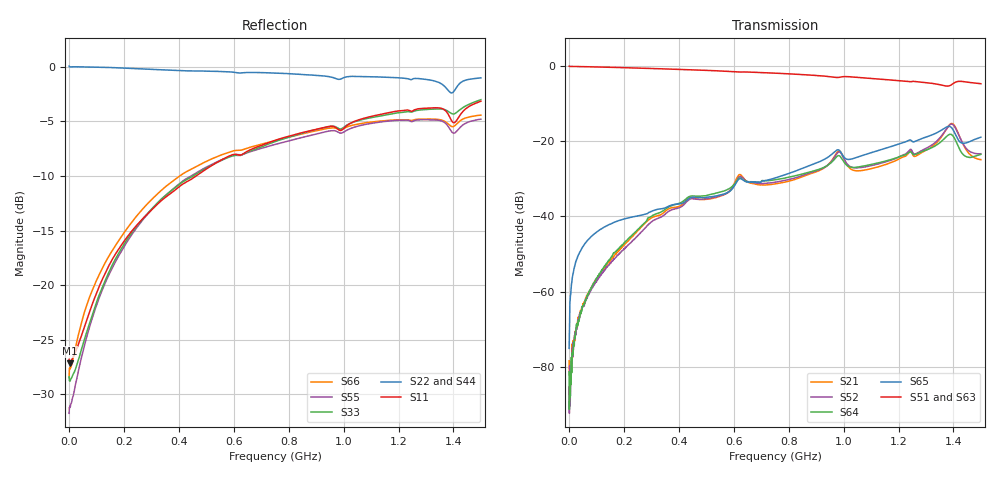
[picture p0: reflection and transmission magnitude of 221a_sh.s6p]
! Generated by Advanced Design System(ADS)'s Touchstone combiner
! Individual SnP file names along with mapping information is saved at the end of this file in XML format
! Created 2019-05-20 11:25:57
# GHz S dB R 50
! 6 Port Network Data
! freq  dBS11  AngS11  dBS12  AngS12  dBS13  AngS13  dBS14  AngS14
!  dBS15  AngS15  dBS16  AngS16
!  dBS21  AngS21  dBS22  AngS22  dBS23  AngS23  dBS24  AngS24
!  dBS25  AngS25  dBS26  AngS26
!  dBS31  AngS31  dBS32  AngS32  dBS33  AngS33  dBS34  AngS34
!  dBS35  AngS35  dBS36  AngS36
!  dBS41  AngS41  dBS42  AngS42  dBS43  AngS43  dBS44  AngS44
!  dBS45  AngS45  dBS46  AngS46
!  dBS51  AngS51  dBS52  AngS52  dBS53  AngS53  dBS54  AngS54
!  dBS55  AngS55  dBS56  AngS56
!  dBS61  AngS61  dBS62  AngS62  dBS63  AngS63  dBS64  AngS64
!  dBS65  AngS65  dBS66  AngS66
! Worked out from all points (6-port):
!   1601 points, 300 kHz to 1.5 GHz, reference 50 ohm
!   strongest paths, dB at 300 kHz, 375.2 MHz, 750.1 MHz, 1.125 GHz, 1.5 GHz:
!     S51: -0.2, -1.0, -2.0, -3.6, -4.8
!     S63: -0.2, -1.0, -2.1, -3.6, -5.1
!     S65: -75.1, -37.0, -29.9, -22.6, -19.0
!     S64: -81.4, -37.1, -30.3, -25.9, -23.6
!     S52: -85.3, -38.3, -31.0, -26.1, -23.4
!     S21: -78.4, -37.7, -31.4, -26.9, -25.0
!   lowest |S11| = -27.2 dB at 2.175 MHz (marker M1), VSWR 1.09, Z = 54.6 - j0.0932 ohm
!   |S11| at or under -10 dB: start of sweep to 462.1 MHz
